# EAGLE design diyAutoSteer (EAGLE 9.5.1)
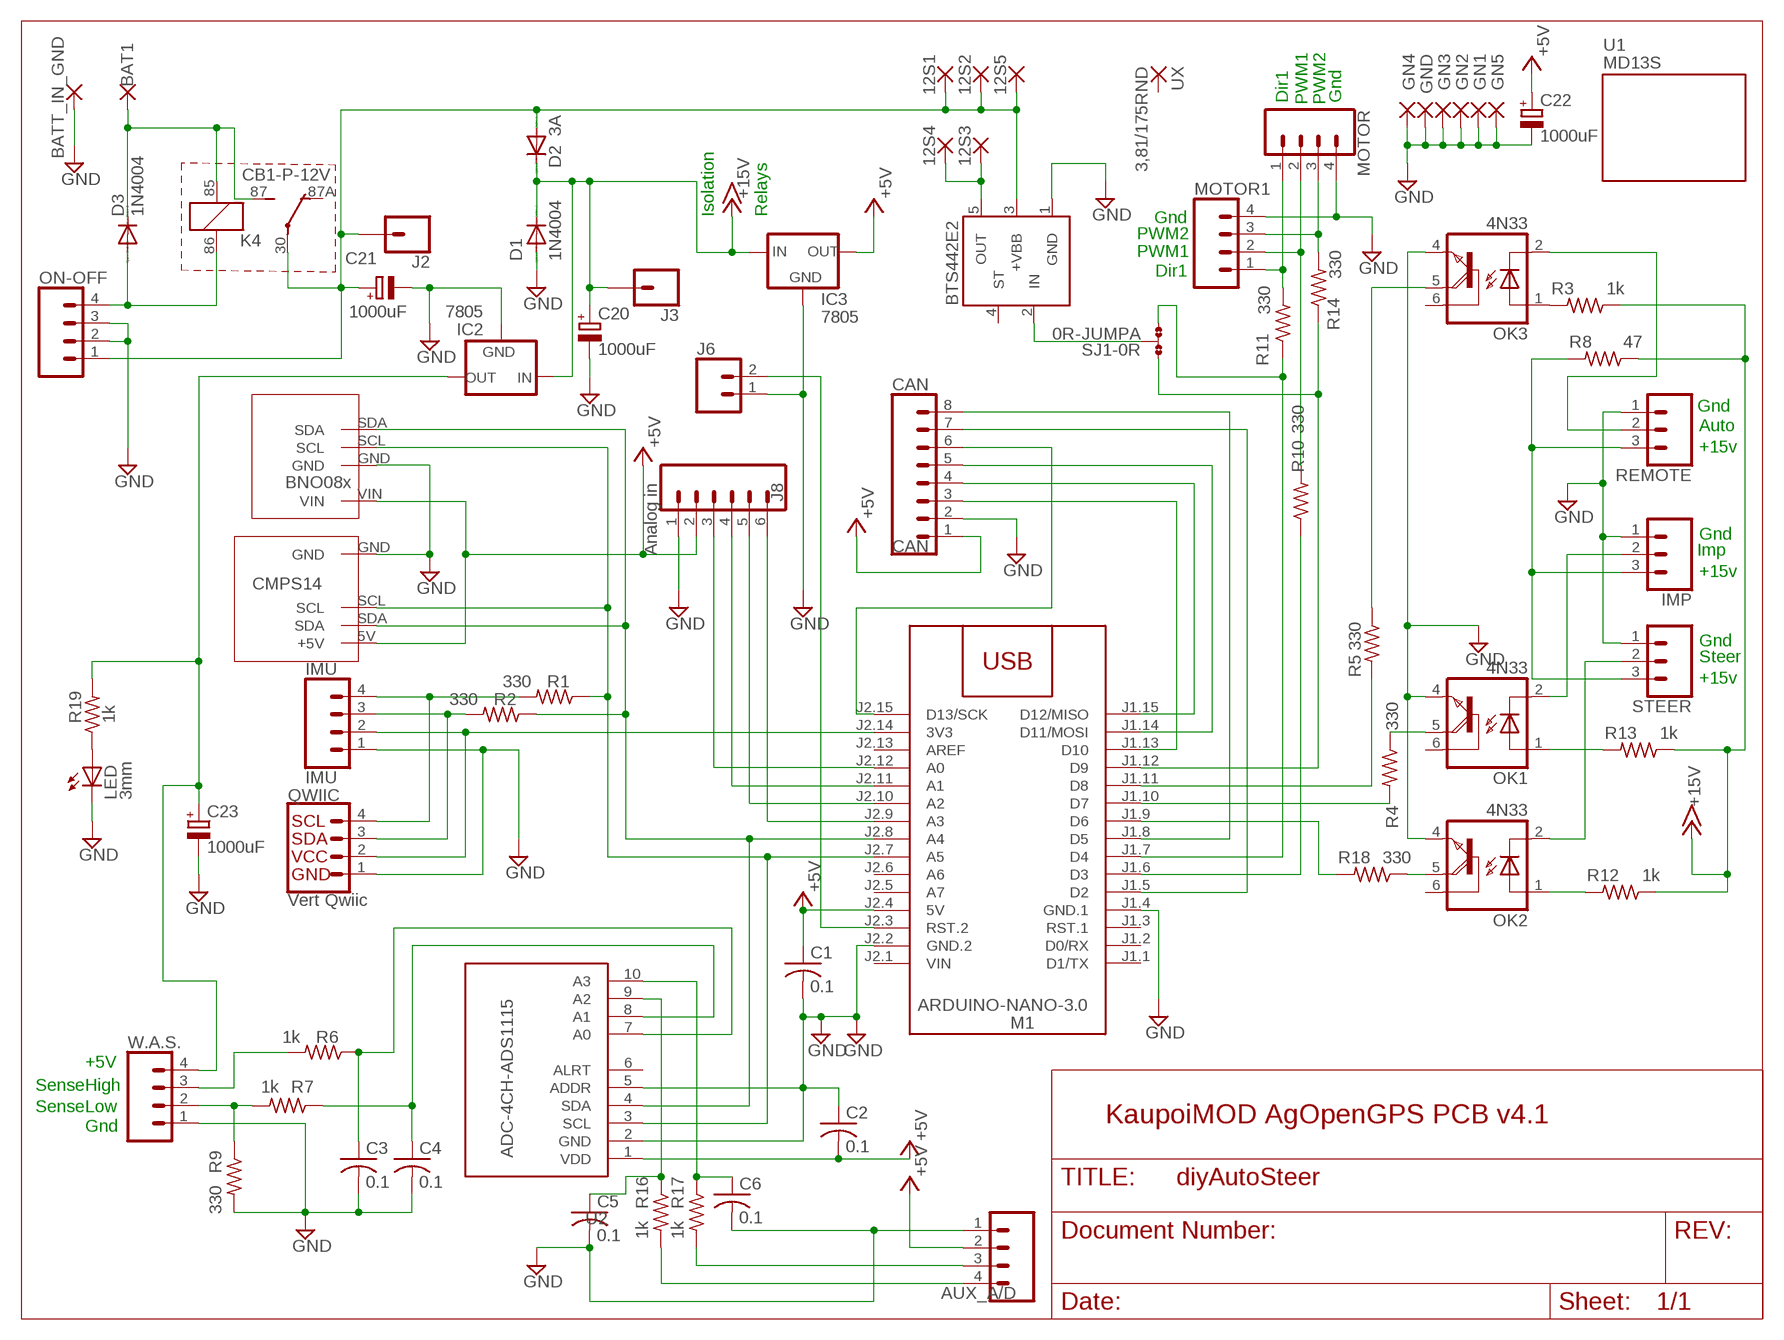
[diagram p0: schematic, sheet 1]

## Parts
12S1  3,81/1,65  [3,81/1,65]
12S2  3,81/1,65  [3,81/1,65]
12S3  3,81/1,65  [3,81/1,65]
12S4  3,81/1,65  [3,81/1,65]
12S5  3,81/1,65  [3,81/1,65]
AUX_A/D  CONN_04LONGPADS  [1X04_LONGPADS]
BAT1  3,81/1,65  [3,81/1,65]
BATT_IN_GND  3,81/1,65  [3,81/1,65]
C1  0.1  C-US025-025X050  [C025-025X050]
C2  0.1  C-US025-025X050  [C025-025X050]
C3  0.1  C-US025-025X050  [C025-025X050]
C4  0.1  C-US025-025X050  [C025-025X050]
C5  0.1  C-US025-025X050  [C025-025X050]
C6  0.1  C-US025-025X050  [C025-025X050]
C20  1000uF  CPOL-EUE5-13  [E5-13]
C21  1000uF  CPOL-EUE5-13  [E5-13]
C22  1000uF  CPOL-EUE5-13  [E5-13]
C23  1000uF  CPOL-EUE5-13  [E5-13]
CAN  CAN  CONN_08NO_SILK_FEMALE_PTH  [1X08_NO_SILK]
D1  1N4004  [DO41-10]
D2  3A  DIODE-DO27-15  [DO27-15]
D3  1N4004  [DO41-10]
GN1  3,81/1,65  [3,81/1,65]
GN2  3,81/1,65  [3,81/1,65]
GN3  3,81/1,65  [3,81/1,65]
GN4  3,81/1,65  [3,81/1,65]
GN5  3,81/1,65  [3,81/1,65]
GND  3,81/1,65  [3,81/1,65]
IC2  7805  78XXS  [78XXS]
IC3  7805  78XXS  [78XXS]
IMP  CONN_03LONGPADS  [1X03_LONGPADS]
IMU  IMU  CONN_04LONGPADS  [1X04_LONGPADS]
J2  CONN_01  [1X01]
J3  CONN_01  [1X01]
J6  CONN_02PTH3  [1X02_LONGPADS]
J8  Analog in  CONN_06NO_SILK_NO_POP  [1X06_NO_SILK]
K4  CB1-P-12V  [CB1]
LED  3mm  LED3MM  [LED3MM]
M1  ARDUINO-NANO-3.0  [ARDUINO-NANO-3.0]
MOTOR  CONN_04LONGPADS  [1X04_LONGPADS]
MOTOR1  CONN_04LONGPADS  [1X04_LONGPADS]
OK1  4N33  [DIL06]
OK2  4N33  [DIL06]
OK3  4N33  [DIL06]
ON-OFF  CONN_04LONGPADS  [1X04_LONGPADS]
QWIIC  Vert Qwiic  QWIIC_CONNECTOR  [JST04_1MM_VERT]
R1  330  R-US_0309/12  [0309/12]
R2  330  R-US_0309/12  [0309/12]
R3  1k  R-US_0309/12  [0309/12]
R4  330  R-US_0309/12  [0309/12]
R5  330  R-US_0309/12  [0309/12]
R6  1k  R-US_0309/12  [0309/12]
R7  1k  R-US_0309/12  [0309/12]
R8  47  R-US_0309/12  [0309/12]
R9  330  R-US_0309/12  [0309/12]
R10  330  R-US_0309/12  [0309/12]
R11  330  R-US_0309/12  [0309/12]
R12  1k  R-US_0309/12  [0309/12]
R13  1k  R-US_0309/12  [0309/12]
R14  330  R-US_0309/12  [0309/12]
R16  1k  R-US_0309/12  [0309/12]
R17  1k  R-US_0309/12  [0309/12]
R18  330  R-US_0309/12  [0309/12]
R19  1k  R-US_0309/12  [0309/12]
REMOTE  CONN_03LONGPADS  [1X03_LONGPADS]
SJ1  0R-JUMPA  [A0R-JMP]
STEER  CONN_03LONGPADS  [1X03_LONGPADS]
U1  MD13S  [MD13S]
U2  ADC-4CH-ADS1115  [ADC-4CH-ADS1115]
U3  BTS442E2  [TO220-5]
U4  CMPS14  [CMPS14]
U5  BNO085  [BNO085]
UX  3,81/175RND  [3,81/1,75RND]
W.A.S.  CONN_04LONGPADS  [1X04_LONGPADS]

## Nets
+5V: AUX_A/D.2 C1.1 C2.2 C22.+ CAN.1 IC3.OUT J8.2 M1.J2.4(5V) U2.1(VDD) U4.5V(+5V) U5.VIN
+15V: C20.+ D1.C D2.C IC2.IN IC3.IN J3.1 R3.1 R8.1 R12.1 R13.1
BATT: BAT1.P$1(P) D3.C K4.85 K4.87(2:S)
DIR: MOTOR1.1 MOTOR.1 R11.2
GND: AUX_A/D.1 BATT_IN_GND.P$1(P) C1.2 C2.1 C3.2 C4.2 C5.2 C6.2 C20.- C21.- C22.- C23.- CAN.2 D1.A GN1.P$1(P) GN2.P$1(P) GN3.P$1(P) GN4.P$1(P) GN5.P$1(P) GND.P$1(P) IC2.GND IC3.GND IMP.1 IMU.1 J6.1 J8.1 LED.K(C) M1.J1.4(GND.1) M1.J2.2(GND.2) MOTOR1.4 MOTOR.4 OK1.4(E) OK2.4(E) OK3.4(E) ON-OFF.2 ON-OFF.3 QWIIC.1 R9.2 REMOTE.1 STEER.1 U2.2(GND) U2.5(ADDR) U3.1(GND) U4.GND U5.GND W.A.S..1
N$1: IMU.2 M1.J2.14(3V3) QWIIC.2
N$2: R7.2 R9.1 W.A.S..2
N$3: IMP.3 R8.2 REMOTE.3 STEER.3
N$4: M1.J1.6(D3) R10.1
N$5: M1.J1.7(D4) R11.1 SJ1.3
N$6: CAN.7 M1.J1.5(D2)
N$7: J6.2 M1.J2.3(RST.2)
N$8: R6.2 W.A.S..3
N$9: CAN.8 M1.J1.8(D5)
N$10: J8.4 M1.J2.11(A1)
N$11: M1.J1.12(D9) R14.1 SJ1.1
N$12: IMU.3 QWIIC.3 R2.2
N$13: IMU.4 QWIIC.4 R1.2
N$14: J8.5 M1.J2.10(A2)
N$15: J8.6 M1.J2.9(A3)
N$16: LED.A R19.1
N$17: CAN.6 M1.J2.15(D13/SCK)
N$18: AUX_A/D.3 R17.2
N$19: OK1.5(COL) R4.1
N$20: C3.1 R6.1 U2.7(A0)
N$21: CAN.5 M1.J1.14(D11/MOSI)
N$22: OK2.2(C) STEER.2
N$23: M1.J1.11(D8) R5.2
N$24: D3.A K4.86 ON-OFF.4
N$25: OK2.1(A) R12.2
N$26: OK3.1(A) R3.2
N$27: M1.J1.10(D7) R4.2
N$28: OK3.2(C) REMOTE.2
N$29: IMP.2 OK1.2(C)
N$30: J8.3 M1.J2.12(A0)
N$31: M1.J1.9(D6) R18.2
N$32: OK1.1(A) R13.2
N$33: CAN.4 M1.J1.15(D12/MISO)
N$34: OK3.5(COL) R5.1
N$35: C6.1 R17.1 U2.10(A3)
N$36: C5.1 R16.1 U2.9(A2)
N$37: CAN.3 M1.J1.13(D10)
N$38: M1.J2.7(A5) R1.1 U2.3(SCL) U4.SCL U5.SCL
N$39: OK2.5(COL) R18.1
N$40: 12S3.P$1(P) 12S4.P$1(P) U3.5(OUT)
N$41: SJ1.2 U3.2(IN)
N$44: C4.1 R7.1 U2.8(A1)
N$47: AUX_A/D.4 R16.2
PWM1: MOTOR1.2 MOTOR.2 R10.2
PWM2: MOTOR1.3 MOTOR.3 R14.2
SDA: M1.J2.8(A4) R2.1 U2.4(SDA) U4.SDA U5.SDA
SW_RAW: 12S1.P$1(P) 12S2.P$1(P) 12S5.P$1(P) C21.+ D2.A J2.1 K4.30(2:P) ON-OFF.1 U3.3(+VBB)
V+WAS: C23.+ IC2.OUT R19.2 W.A.S..4
Unconnected: K4.87A(2:O) M1.J1.1(D1/TX) M1.J1.2(D0/RX) M1.J1.3(RST.1) M1.J2.5(A7) M1.J2.6(A6) M1.J2.13(AREF) OK1.6(B) OK2.6(B) OK3.6(B) U2.6(ALRT) U3.4(ST) UX.P$1(P)

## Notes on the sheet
- Dir1 | PWM1 | PWM2 | Gnd
- Gnd
- Isolation | Relays
- PWM2
- PWM1
- Dir1
- Gnd
- Auto
- +15v
- Gnd
- Imp
- +15v
- Gnd
- Steer
- +15v
- +5V
- Sense | High
- Sense | Low
- KaupoiMOD AgOpenGPS PCB v4.1
- Gnd

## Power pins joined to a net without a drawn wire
VIN: M1.J2.1(VIN)

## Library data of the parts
12S1-12S5 BAT1 BATT_IN_GND GN1-GN5 GND = wirepad:3,81/1,65: 3,81/1,65
AUX_A/D IMU MOTOR MOTOR1 ON-OFF W.A.S. = SparkFun-Connectors:CONN_04: Multi connection point. Often used as Generic Header-pin footprint for 0.1 inch spaced/style header connections On any of the 0.1 inch spaced packages, you can populate with these: Break Away Headers - Straight (PRT-00116) Break Away Male Headers - Right Angle (PRT-00553) Female Headers (PRT-00115)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; PROD_ID: CONN-09696
C1-C6 = rcl:C-US: CAPACITOR, American symbol
C20 = rcl:CPOL-EU: POLARIZED CAPACITOR, European symbol; SPICEPREFIX: C
C21-C23 = rcl:CPOL-EU: POLARIZED CAPACITOR, European symbol
CAN = SparkFun-Connectors:CONN_08: Multi connection point. Often used as Generic Header-pin footprint for 0.1 inch spaced/style header connections On any of the 0.1 inch spaced packages, you can populate with these: Break Away Headers - Straight (PRT-00116) Break Away Male Headers - Right Angle (PRT-00553) Female Headers (PRT-00115)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; PROD_ID: CONN-08438
D1 D3 = diode:1N4004: DIODE
D2 = diode:DIODE-: DIODE
IC2 IC3 = v-reg:78XXS: VOLTAGE REGULATOR
IMP REMOTE STEER = SparkFun-Connectors:CONN_03: Multi connection point. Often used as Generic Header-pin footprint for 0.1 inch spaced/style header connections On any of the 0.1 inch spaced packages, you can populate with these: Break Away Headers - Straight (PRT-00116) Break Away Male Headers - Right Angle (PRT-00553) Female Headers (PRT-00115)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
J2 J3 = SparkFun-Connectors:CONN_01: Single connection point. Often used as Generic Header-pin footprint for 0.1 inch spaced/style header connections
J6 = SparkFun-Connectors:CONN_02: Multi connection point. Often used as Generic Header-pin footprint for 0.1 inch spaced/style header connections
J8 = SparkFun-Connectors:CONN_06: Multi connection point. Often used as Generic Header-pin footprint for 0.1 inch spaced/style header connections On any of the 0.1 inch spaced packages, you can populate with these: Break Away Headers - Straight (PRT-00116) Break Away Male Headers - Right Angle (PRT-00553) Female Headers (PRT-00115)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
K4 = relay:CB1*: HIGH POWER AUTOMOTIVE RELAY Form C NAiS Source: http://www.mew-europe.com/.. en_ds_61202_0000.pdf; MF: AROMAT/ MATSUSHITA; MPN: CB1-P-12V; OC_FARNELL: unknown; OC_NEWARK: 52F9201
LED = led:LED: LED
M1 = diy-modules:ARDUINO-NANO-3.0: Arduino Nano 3.0 and compatible devices More details available here: https://www.arduino.cc/en/Main/ArduinoBoardNano Click here to find device on ebay.com
OK1-OK3 = optocoupler:4N33: MOTOROLA OPTO COUPLER; MF: VISHAY/TELEFUNKEN; MPN: 4N33; OC_FARNELL: 1469601; OC_NEWARK: 88K1390
QWIIC = SparkFun-Connectors:QWIIC_CONNECTOR: SparkFun I2C Standard Qwiic Connector An SMD 1mm pitch JST connector makes it easy and quick (get it? Qwiic?) to connect I2C devices to each other. The Qwiic system enables fast and solderless connection between popular platforms and various sensors and actuators. We carry 200mm, 100mm, 50mm, and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; PROD_ID: CONN-14483; VALUE: Vertical Qwiic Connector
R1-R14 R16-R19 = rcl:R-US_: RESISTOR, American symbol
SJ1 = jump-0r-smd:0R-JUMP: SMD 0R 0805 Jumper
U1 = cytronMD13Sholes:MD13S: 13Amp DC Motor Driver (MD13S); CYTRON-PC: MD13S; DESC: 13Amp DC Motor Driver - GROVE Compatible; MF: Cytron; MPN: MD13S
U2 = diy-modules:ADC-4CH-ADS1115: 4 Channel 16-Bit Analog-to-Digital Converter based on ADS1115 chip Arduino ADS1115 Getting Started Tutorial is available here: http://henrysbench.capnfatz.com/henrys-bench/arduino-voltage-measurements/arduino-ads1115-module-getting-started-tutorial/ ADS1115 datasheet is available here: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
U3 = v-reg-3:BTS442E2
U4 = IMU:CMPS14: CMPS14
U5 = IMU:BNO085
UX = wirepad:3,81/175RND

## Module MOTOR_CONTROLLER
Ports: 

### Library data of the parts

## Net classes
0 default: clearance 0.205 mm

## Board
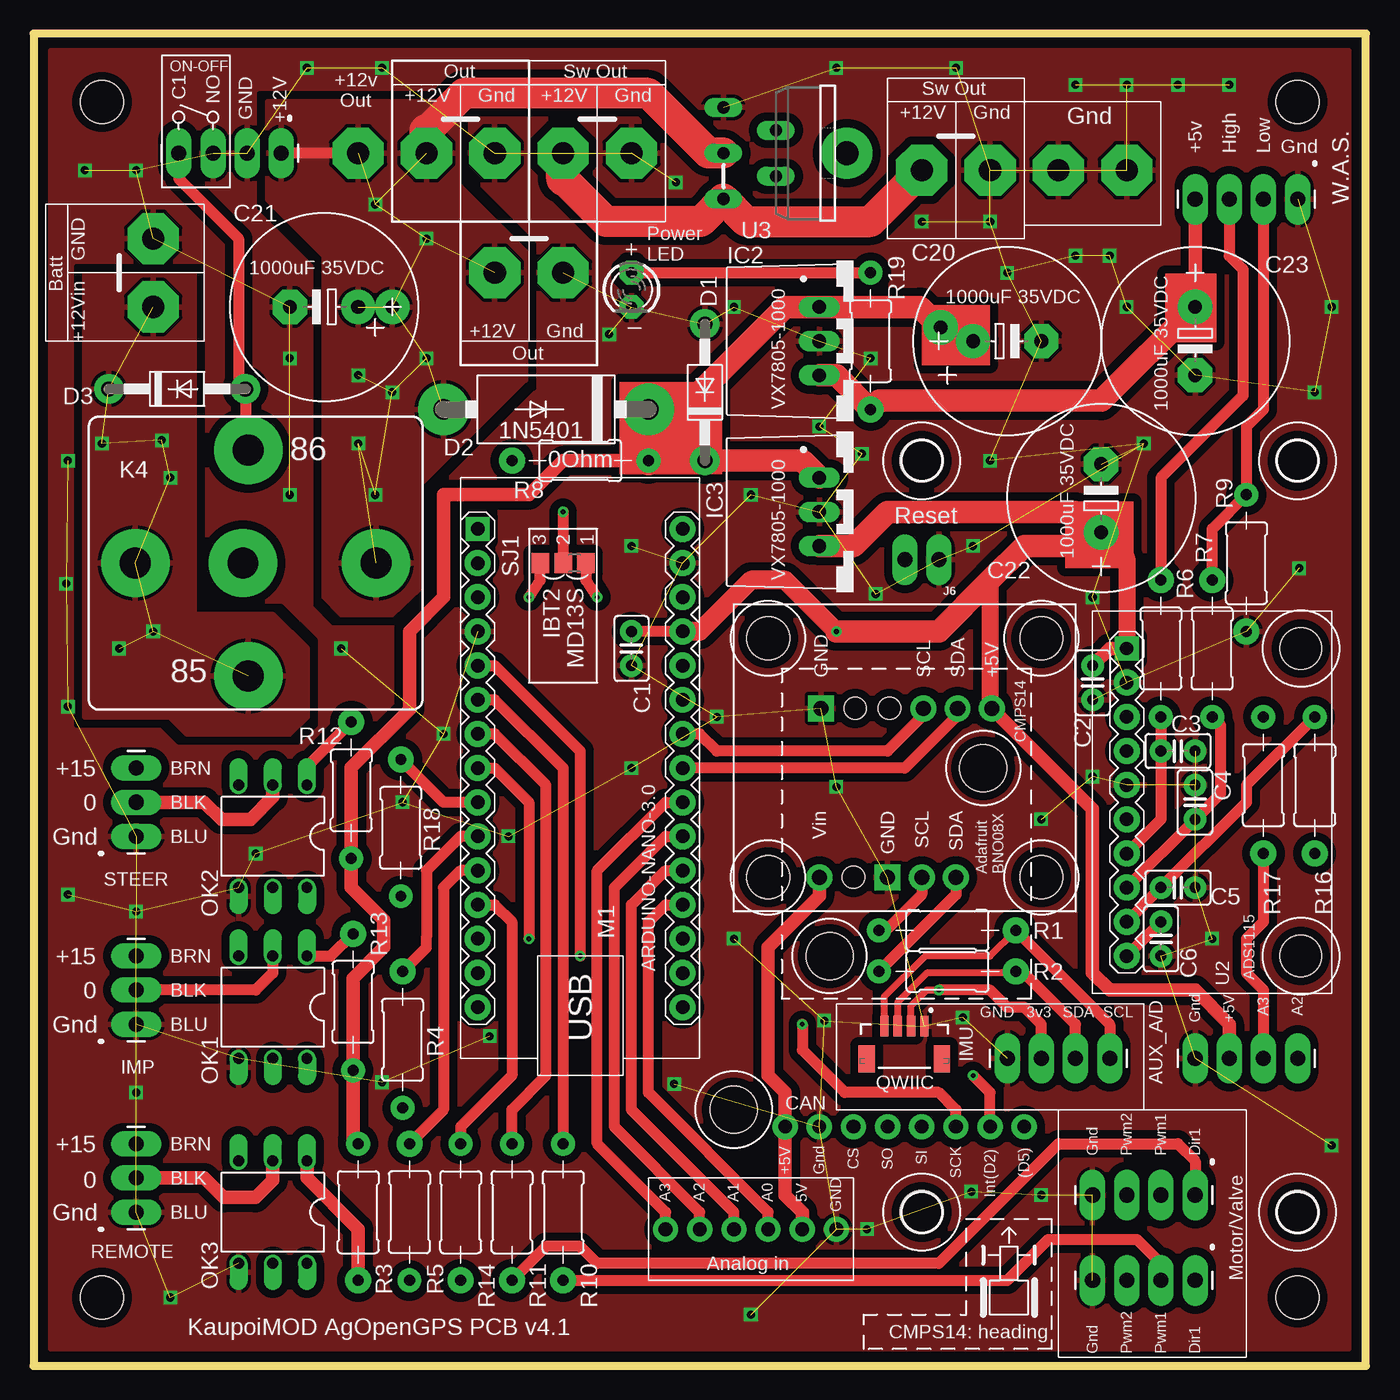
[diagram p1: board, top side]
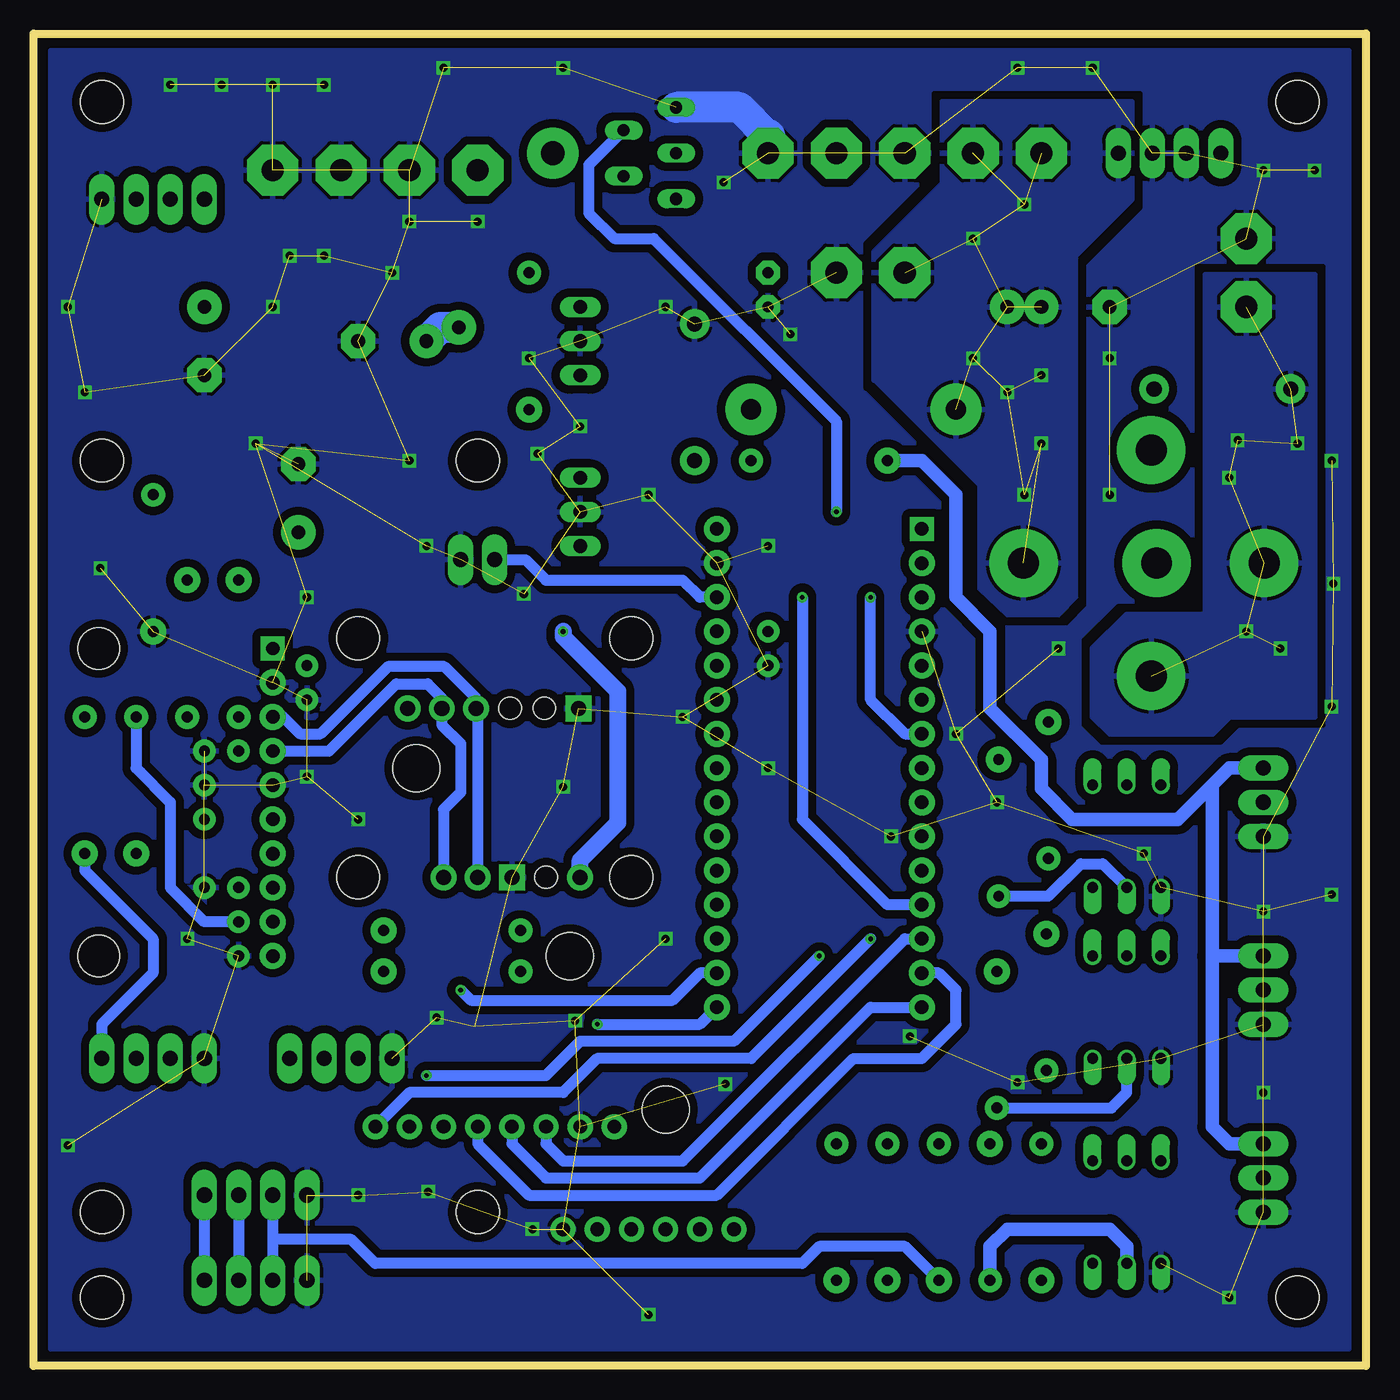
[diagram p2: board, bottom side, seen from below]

Size 99.06 x 99.06 mm. Coordinates in mm from the lower left corner, seen from the top.
Outline: 0,0 99.06,0 99.06,99.06 0,99.06 0,0
Copper layers (1*16): Top 0.035mm / dielectric 1.5mm / Bottom 0.035mm
Design rules "default *": minimum track width 16mil, minimum drill 0.35mm, track to track 6mil, track to pad 6mil, pad to pad 6mil, via to via 6mil, smd to smd 6mil, copper to edge 8mil, drill to drill 6mil, minimum pad ring 10mil, minimum via ring 8mil, stop-mask expansion 4mil, vias tented up to drill 0mil, thermal gap 10mil
Holes 3.2 mm at 5.08,5.08 93.98,5.08 5.08,93.98 93.98,93.98
Holes 3.5 mm at 52.07,19.05

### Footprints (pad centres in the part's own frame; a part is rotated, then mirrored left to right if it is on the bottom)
3,81/1,65 = drill 1.651 pad 3.81 octagon: P$1 0,0
1X04_LONGPADS = drill 1.118 pad 1.88 long: 1 0,0; 2 2.54,0; 3 5.08,0; 4 7.62,0
C025-025X050 = drill 0.813 pad 1.676: 1 -1.27,0; 2 1.27,0
E5-13 = drill 1.016 pad 2.54: + -2.54,0 | drill 1.016 pad 2.54 octagon: - 2.54,0
1X08_NO_SILK = drill 1.016 pad 1.88: 1 0,0; 2 2.54,0; 3 5.08,0; 4 7.62,0; 5 10.16,0; 6 12.7,0; 7 15.24,0; 8 17.78,0
DO41-10 = drill 1.118 pad 2.184: A 5.08,0; C -5.08,0
DO27-15 = drill 1.499 pad 3.81: A 7.62,0; C -7.62,0
78XXS = drill 1.016 long: GND 0,-2.54; IN -2.54,-2.54; OUT 2.54,-2.54
1X03_LONGPADS = drill 1.118 pad 1.88 long: 1 0,0; 2 2.54,0; 3 5.08,0
1X01 = drill 1.016 pad 2.54: 1 0,0
1X02_LONGPADS = drill 1.118 pad 1.88 long: 1 0,0; 2 2.54,0
1X06_NO_SILK = drill 1.016 pad 1.88: 1 0,0; 2 2.54,0; 3 5.08,0; 4 7.62,0; 5 10.16,0; 6 12.7,0
CB1 = drill 2.3 pad 5.08: 30 8.95,0; 85 -0.55,-8.4; 86 -0.55,8.4; 87 -8.95,0; 87A -0.95,0
LED3MM = drill 0.813 pad 1.778 octagon: A -1.27,0; K 1.27,0
ARDUINO-NANO-3.0 = drill 1 pad 1.778 square: J1.1 17.78,7.62 | drill 1 pad 1.93: J1.2 15.24,7.62; J1.3 12.7,7.62; J1.4 10.16,7.62; J1.5 7.62,7.62; J1.6 5.08,7.62; J1.7 2.54,7.62; J1.8 0,7.62; J1.9 -2.54,7.62; J1.10 -5.08,7.62; J1.11 -7.62,7.62; J1.12 -10.16,7.62; J1.13 -12.7,7.62; J1.14 -15.24,7.62; J1.15 -17.78,7.62; J2.1 17.78,-7.62; J2.2 15.24,-7.62; J2.3 12.7,-7.62; J2.4 10.16,-7.62; J2.5 7.62,-7.62; J2.6 5.08,-7.62; J2.7 2.54,-7.62; J2.8 0,-7.62; J2.9 -2.54,-7.62; J2.10 -5.08,-7.62; J2.11 -7.62,-7.62; J2.12 -10.16,-7.62; J2.13 -12.7,-7.62; J2.14 -15.24,-7.62; J2.15 -17.78,-7.62
DIL06 = drill 0.813 offset: 1 -2.54,-3.81; 2 0,-3.81; 3 2.54,-3.81; 4 2.54,3.81; 5 0,3.81; 6 -2.54,3.81
JST04_1MM_VERT = smd 0.6 x 1.55: 1 -1.478,0.775; 2 -0.478,0.775; 3 0.522,0.775; 4 1.522,0.775 | smd 1.2 x 2: NC1 -2.778,3.2; NC2 2.822,3.2
0309/12 = drill 0.813 pad 1.778: 1 -5.08,0 | drill 0.813 pad 1.93: 2 5.08,0
A0R-JMP = smd 1.5 x 1.3: 1 0,1.7; 2 0,0; 3 0,-1.7
MD13S = hole 3.2: 2.54,30.48; 2.54,2.54; 58.42,2.54; 58.42,30.48
ADC-4CH-ADS1115 = drill 1 pad 1.778 square: 1 -6.35,11.43 | drill 1 pad 1.93: 2 -6.35,8.89; 3 -6.35,6.35; 4 -6.35,3.81; 5 -6.35,1.27; 6 -6.35,-1.27; 7 -6.35,-3.81; 8 -6.35,-6.35; 9 -6.35,-8.89; 10 -6.35,-11.43 | hole 3.1: 6.604,11.43; 6.604,-11.43
TO220-5 = drill 0.9 long: 1 -3.4,-8.4; 2 -1.7,-4.5; 3 0,-8.4; 4 1.7,-4.5; 5 3.4,-8.4
CMPS14 = drill 1.118 pad 1.93: 5V 10.16,-6.35; SCL 10.16,-1.27; SDA 10.16,-3.81 | drill 1.118 pad 1.93 square: GND 10.16,6.35 | hole 3.5: 5.715,-5.715; -8.255,5.715 | hole 1.676: 10.16,1.27; 10.16,3.81
BNO085 = drill 1.118 pad 1.93 square: GND 8.89,-1.27 | drill 1.118 pad 1.93: SCL 8.89,1.27; SDA 8.89,3.81; VIN 8.89,-6.35 | hole 3.2: 8.89,10.16; 8.89,-10.16; -8.89,-10.16; -8.89,10.16 | hole 1.651: 8.89,-3.81
3,81/1,75RND = drill 1.75 pad 3.81: P$1 0,0

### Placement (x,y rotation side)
12S1  29.21,90.17 0 top
12S2  24.13,90.17 0 top
12S3  39.37,90.17 0 top
12S4  66.04,88.9 0 top
12S5  34.29,81.28 0 top
AUX_A/D  86.36,22.86 0 top
BAT1  8.89,78.74 0 top
BATT_IN_GND  8.89,83.82 0 top
C1  44.45,53.34 270 top
C2  78.74,50.8 90 top
C3  85.09,45.72 0 top
C4  86.36,41.91 90 top
C5  85.09,35.56 0 top
C6  83.82,31.75 270 top
C20  72.39,76.2 0 top
C21  21.59,78.74 180 top
C22  79.38,64.52 90 top
C23  86.36,76.2 270 top
CAN  55.88,17.78 0 top
D1  49.91,72.39 90 top
D2  38.1,71.12 180 top
D3  10.67,72.64 0 top
GN1  34.29,90.17 0 top
GN2  71.12,88.9 0 top
GN3  81.28,88.9 0 top
GN4  44.45,90.17 0 top
GN5  39.37,81.28 0 top
GND  76.2,88.9 0 top
IC2  60.96,76.2 270 top
IC3  60.96,63.5 270 top
IMP  7.62,25.4 90 top
IMU  72.39,22.86 0 top
J2  26.67,78.74 0 top
J3  67.44,77.22 0 top
J6  67.31,59.94 180 top
J8  59.69,10.16 180 top
K4  16.51,59.69 0 top
LED  44.45,80.01 270 top
M1  40.64,44.45 90 top
MOTOR  86.36,6.35 180 top
MOTOR1  86.36,12.7 180 top
OK1  17.78,26.67 180 top
OK2  17.78,39.37 180 top
OK3  17.78,11.43 180 top
ON-OFF  18.41,90.17 180 top
QWIIC  64.77,26.04 180 top
R1  67.95,32.38 0 top
R2  67.95,29.34 0 top
R3  24.13,11.43 270 top
R4  27.43,24.26 90 top
R5  27.94,11.43 90 top
R6  83.82,53.34 90 top
R7  87.63,53.34 90 top
R8  40.64,67.31 180 top
R9  90.17,59.69 270 top
R10  39.37,11.43 270 top
R11  35.56,11.43 270 top
R12  23.62,42.8 90 top
R13  23.75,27.05 90 top
R14  31.75,11.43 270 top
R16  95.25,43.18 270 top
R17  91.44,43.18 270 top
R18  27.3,40.01 90 top
R19  62.23,76.2 270 top
REMOTE  7.62,11.43 90 top
SJ1  39.37,59.69 270 top
STEER  7.62,39.37 90 top
U1  96.52,8.89 90 top
U2  87.63,41.91 0 top
U3  59.69,90.17 270 top
U4  64.9,38.73 90 top
U5  64.77,45.21 270 top
UX  60.45,90.17 0 top
W.A.S.  93.98,86.74 180 top

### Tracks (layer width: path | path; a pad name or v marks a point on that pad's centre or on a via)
+5V  (via drill 0.35)
  Top 0.813: M1.J2.4 C1.1
  Top 1.016: U2.1 80.01,53.34 C2.2 | U4.5V 78.74,41.4 78.74,29.21 80.01,27.94 86.36,27.94 88.9,25.4 AUX_A/D.2 | U5.VIN 58.42,34.92 54.61,31.11 54.61,21.59 55.88,20.32 CAN.1 55.88,12.7 57.15,11.43 J8.2
  Top 1.27: C22.+ 81.28,60.07 U2.1 | 71.12,58.42 71.12,49.02 U4.5V
  Top 1.422: v59.69,54.61 55.88,58.42 53.34,58.42 49.53,54.61 M1.J2.4
  Top 1.676: v59.69,54.61 67.31,54.61 71.12,58.42 73.66,60.96 78.36,60.96 C22.+ 78.99,61.98 77.47,63.5 63.5,63.5 60.96,60.96 IC3.OUT
  Bottom 1.27: v59.69,54.61 59.69,54.23 55.63,50.16 55.63,40.39 58.42,37.59 U5.VIN
+15V
  Top 1.016: R3.1 23.75,16.89 R13.1 23.75,28.83 26.04,31.11 26.04,33.15 23.62,35.56 R12.1 23.62,44.49 27.94,48.81 27.94,54.61 30.48,57.15 30.48,64.77 30.49,64.78 36.84,64.78 39.37,67.31 R8.1 49.53,66.93 D1.C
  Top 1.676: D2.C 45.8,71.2 48.34,71.2 55.88,78.74 IC2.IN 65.91,78.74 J3.1 | R8.1 57.15,67.31 IC3.IN
  Top 2.184: R8.1 D2.C
  Bottom 2.286: J3.1 68.83,77.22 C20.+
BATT  (via drill 0.6)  (8 unrouted)
  other vias: 9.53,68.83 5.08,68.58 8.89,54.61 10.16,66.04 6.35,53.34
  pour Bottom (isolate 0.406): 19.05,46.99 20.32,48.26 20.32,53.34 17.78,55.88 11.94,55.88 11.94,81.15 3.81,81.15 3.81,48.26 10.16,48.26 11.43,46.99
  pour Top (isolate 0.406): 3.81,81.15 3.81,48.26 10.16,48.26 11.43,46.99 19.05,46.99 20.32,48.26 20.32,53.34 17.78,55.88 11.94,55.88 11.94,81.15
DIR
  Top 0.813: R11.2 38.1,8.89 40.64,8.89 41.91,7.62 67.31,7.62 76.2,16.51 85.09,16.51 86.36,15.24 MOTOR1.1
  Bottom 0.813: MOTOR1.1 MOTOR.1
GND  (via drill 0.6)  (107 unrouted)
  Bottom 2.286: 44.45,91.44 46.58,93.57 U3.1
  Bottom 2.54: GN4.P$1 44.45,91.44
  other vias: 20.32,96.52 7.62,88.9 42.8,76.71 59.69,96.52 96.52,78.74 47.75,88.01 88.9,95.25 33.91,24.51 81.28,78.74 95.25,72.39 62.23,74.93 61.59,67.82 58.42,69.85 53.34,64.77 27.43,41.91 30.48,46.99 52.07,78.74 66.04,85.09 72.39,81.28 71.12,85.09 77.47,82.55 2.54,67.31 2.54,49.02 7.62,20.32 94.11,59.31 53.34,3.81 47.62,20.95 78.74,57.15 69.09,25.91 3.81,88.9 25.91,96.52 19.05,74.93 19.05,64.77 22.86,53.34 2.41,58.17 7.62,33.78 16.51,38.1 69.85,60.96 81.28,95.25 44.45,44.45 44.45,60.96 85.09,95.25 80.01,82.55 62.61,57.4 71.12,67.31 96.52,16.38 69.72,12.95 78.74,43.81 10.16,5.08 52.07,31.75 82.55,68.58 59.69,43.05 50.8,48.26 87.63,31.75 61.98,10.16 2.54,35.05 77.47,95.25 74.93,12.7 25.91,21.08 58.8,25.65 74.93,40.64 68.58,96.52 35.31,39.37
  pour Bottom (isolate 0.61, rank 2): 1.27,97.79 1.27,1.27 97.79,1.27 97.79,97.79
  pour Top (isolate 0.61, rank 2): 1.27,97.79 1.27,1.27 97.79,1.27 97.79,97.79
N$1  (via drill 0.35)
  Top 0.508: QWIIC.2 65.25,26.77 66.42,27.94 v67.31,27.94
  Top 0.813: IMU.2 74.93,25.4 73.66,26.67 72.39,26.67 71.12,27.94 v67.31,27.94
  Bottom 0.813: M1.J2.14 49.53,29.21 51.56,27.18 66.55,27.18 v67.31,27.94
N$2
  Top 0.813: R7.2 87.63,62.23 R9.1 90.17,69.85 91.44,71.12 W.A.S..2
N$3
  Bottom 1.016: 11.43,43.18 10.16,44.45 STEER.3 | 11.43,43.18 11.43,30.48 | IMP.3 11.43,30.48 | 11.43,30.48 11.43,17.78 10.16,16.51 REMOTE.3 | 11.43,43.18 13.97,40.64 21.84,40.64 24.13,42.93 24.13,45.09 27.94,48.9 27.94,54.61 30.48,57.15 30.48,64.77 33.02,67.31 R8.2
N$4
  Top 0.813: R10.1 39.37,44.45 34.29,49.53 M1.J1.6
N$5  (via drill 0.35)
  Top 0.813: R11.1 35.56,19.05 38.1,21.59 38.1,43.18 34.29,46.99 M1.J1.7 | SJ1.3 37.67,58.42 v36.83,57.15
  Bottom 0.813: M1.J1.7 34.29,46.99 36.83,49.53 v36.83,57.15
N$6  (via drill 0.35)
  Top 0.813: M1.J1.5 34.29,52.07 40.64,45.72 v40.64,30.48 | CAN.7 71.12,20.32 v69.85,21.59
  Bottom 0.813: v40.64,30.48 46.99,24.13 58.42,24.13 60.96,21.59 v69.85,21.59
N$7
  Bottom 0.813: J6.2 62.48,59.94 60.96,58.42 50.8,58.42 49.53,57.15 M1.J2.3
N$8
  Top 0.813: R6.2 83.82,66.04 89.92,72.14 89.92,81.53 88.9,82.55 W.A.S..3
N$9  (via drill 0.35)
  Top 0.813: M1.J1.8 34.29,44.45 36.83,41.91 v36.83,31.75
  Bottom 0.813: v36.83,31.75 45.72,22.86 57.15,22.86 59.69,20.32 71.12,20.32 CAN.8
N$10
  Top 0.813: J8.4 52.07,11.43 44.45,19.05 44.45,34.29 46.99,36.83 M1.J2.11
N$11  (via drill 0.35)
  Top 0.813: M1.J1.12 34.29,34.29 35.56,33.02 35.56,21.59 31.75,17.78 R14.1 | SJ1.1 41.07,58.42 v41.91,57.15
  Bottom 0.813: v41.91,57.15 41.91,40.64 35.56,34.29 M1.J1.12
N$12
  Top 0.508: R2.2 72.9,29.21 66.42,29.21 64.23,27.02 64.23,25.27 QWIIC.3
  Top 0.813: IMU.3 77.47,25.4 73.53,29.34 R2.2
N$13
  Top 0.508: QWIIC.4 63.23,25.27 63.23,27.42 66.29,30.48 71.12,30.48 R1.2
  Top 0.813: R1.2 80.01,25.4 80,22.87 IMU.4
N$14
  Top 0.813: J8.5 49.53,11.43 43.18,17.78 43.18,35.56 46.99,39.37 M1.J2.10
N$15
  Top 0.813: J8.6 46.99,11.43 41.91,16.51 41.91,36.83 46.99,41.91 M1.J2.9
N$16
  Top 0.813: LED.A R19.1
N$17  (via drill 0.35)
  Top 0.813: CAN.6 68.58,19.05 67.31,20.32 60.32,20.32 57.15,23.5 v57.15,25.4
  Bottom 0.813: M1.J2.15 49.53,25.4 v57.15,25.4
N$18
  Top 0.813: R17.2 91.44,33.02 90.17,31.75 90.17,29.21 91.44,27.94 AUX_A/D.3
N$19
  Bottom 0.813: R4.1 18.92,19.18 17.78,20.32 OK1.5
N$20
  Top 0.813: U2.7 83.82,40.64 C3.1 R6.1
N$21
  Bottom 0.813: CAN.5 66.04,16.51 62.23,12.7 48.26,12.7 38.1,22.86 33.02,22.86 30.48,25.4 30.48,27.94 31.75,29.21 M1.J1.14
N$22
  Top 1.016: OK2.2 17.78,42.29 16.13,40.64 13.97,40.64 12.7,41.91 STEER.2
N$23
  Top 0.813: M1.J1.11 31.75,36.83 30.48,35.56 30.48,19.05 R5.2
N$24
  Top 0.813: K4.86 15.75,68.3 D3.A 15.24,73.15 15.24,83.82 10.79,88.27 ON-OFF.4
N$25
  Top 0.813: R12.2 20.32,44.58 OK2.1
N$26
  Top 1.016: OK3.1 20.32,13.97 24.13,10.16 R3.2
N$27
  Top 0.813: M1.J1.10 31.75,39.37 29.21,36.83 29.21,31.88 29.21,31.11 R4.2
N$28
  Top 1.016: OK3.2 17.78,13.79 16.5,12.52 14.14,12.53 12.7,13.97 REMOTE.2
N$29
  Top 0.813: OK1.2 17.78,29.21 16.51,27.94 IMP.2
N$30
  Top 0.813: J8.3 54.61,11.43 45.72,20.32 45.72,33.02 46.99,34.29 M1.J2.12
N$31
  Top 0.813: M1.J1.9 30.48,41.91 R18.2
N$32
  Top 0.813: OK1.1 22.1,30.48 R13.2
N$33
  Bottom 0.813: CAN.4 63.5,16.51 60.96,13.97 49.53,13.97 36.83,26.67 M1.J1.15
N$34
  Bottom 1.016: R5.1 27.94,8.89 26.67,10.16 19.05,10.16 17.78,8.89 OK3.5
N$35
  Top 0.813: C6.1 U2.10
  Bottom 0.813: R17.1 91.44,44.45 88.9,41.91 88.9,35.56 86.36,33.02 C6.1
N$36
  Top 0.813: U2.9 C5.1 90.17,41.91 90.17,43.18 R16.1
N$37
  Bottom 0.813: M1.J1.13 34.29,31.75 50.8,15.24 59.69,15.24 60.96,16.51 CAN.3
N$38
  Top 0.813: U4.SCL 66.17,48.39 63.5,45.72 50.8,45.72 49.53,46.99 M1.J2.7 | U5.SCL 66.04,35.05 63.37,32.38 R1.1
  Bottom 0.813: U2.3 80.52,48.26 79.25,46.99 77.72,46.99 72.72,52 68.51,52 66.17,49.66 U4.SCL 66.04,48.77 U5.SCL
N$39
  Bottom 0.813: OK2.5 19.56,37.34 21.21,37.34 23.62,34.92 R18.1
N$40
  Top 2.286: 39.37,88.27 42.54,85.09 49.61,85.09 U3.5 52.97,85.09 62.23,85.09 12S4.P$1
  Top 2.54: 39.37,88.27 12S3.P$1
N$41  (via drill 0.35)
  Top 0.813: v39.37,63.5 SJ1.2
  Bottom 0.813: U3.2 57.78,89.28 57.78,85.72 55.88,83.82 52.96,83.82 39.37,70.23 v39.37,63.5
N$44
  Top 0.813: U2.8 C4.1 88.27,42.55 88.27,47.62 R7.1
N$47
  Bottom 0.813: R16.2 95.25,36.83 90.17,31.75 90.17,29.21 93.98,25.4 AUX_A/D.4
PWM1
  Top 0.813: R10.2 72.39,6.35 75.44,9.4 82.04,9.4 83.82,7.62 MOTOR.2
  Bottom 0.813: MOTOR1.2 MOTOR.2
PWM2
  Bottom 0.813: MOTOR1.3 MOTOR.3 81.28,9.4 75.44,9.4 73.66,7.62 41.91,7.62 40.64,8.89 34.29,8.89 R14.2
SDA
  Top 0.813: U4.SDA 68.71,48.39 64.77,44.45 M1.J2.8 | U5.SDA 68.58,35.05 R2.1
  Bottom 0.813: U2.4 77.09,45.72 72.09,50.72 69.77,50.72 68.71,49.66 U4.SDA 68.71,47.66 67.31,46.26 67.31,42.64 68.58,41.37 U5.SDA
SW_RAW  (via drill 0.6)  (13 unrouted)
  Top 0.813: 12S2.P$1 ON-OFF.1
  Top 2.286: U3.3 50.16,90.17 45.72,94.61 32,94.61 29.21,91.82
  Top 2.54: 12S1.P$1 29.21,91.82
  other vias: 25.4,86.36 29.21,83.82 26.67,72.39 29.21,74.93 25.4,64.77 24.13,73.66 24.13,68.58
  pour Bottom (isolate 0.406): 17.4,93.98 17.4,86.74 21.59,82.55 21.59,57.15 22.86,55.88 26.67,55.88 28.7,57.78 28.7,65.53 36.45,73.28 36.58,73.28 36.58,82.8 31.5,87.88 31.5,93.98
  pour Top (isolate 0.406): 17.4,93.98 17.4,86.74 21.59,82.55 21.59,57.15 22.86,55.88 26.67,55.88 28.7,57.78 28.7,65.53 36.45,73.28 36.58,73.28 36.58,82.8 31.5,87.88 31.5,93.98
V+WAS
  Top 1.016: W.A.S..4 C23.+
  Top 1.676: IC2.OUT 59.69,73.66 R19.2 62.87,71.75 79.38,71.75 C23.+
(copper drawn outside any net)
  shapes: Top area x4

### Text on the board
tPlace: C1 | NO | GND | +12V | Out | Sw Out | +12v / Out | +12V | Gnd | +12V | Gnd | Sw Out | +12V | Gnd | Gnd | +5v | High | Low | Gnd | C21 | + | _ | +12Vin | +12V | Gnd | Out | Reset | 3 | 2 | 1 | IBT2 ( | MD13S ( | +15 | BRN | BLK | 0 | Gnd | BLU | +15 | BRN | BLK | 0 | GND | 3v3 | SDA | SCL | Gnd | +5V | A3 | A2 | Gnd | BLU | BRN | +15 | Int(D2) | Gnd | Pwm2 | Pwm1 | Dir1 | CS | SO | SI | BLK | +5V | Gnd | SCK | (D5) | 0 | A3 | A2 | A1 | A0 | 5V | Gnd | BLU | GND | Analog in | Motor/Valve | KaupoiMOD AgOpenGPS PCB v4.1 | Gnd | Pwm2 | Pwm1 | Dir1
tNames: GND | 1000uF 35VDC | Power / LED | Batt | 1000uF 35VDC | VX7805-1000 | 1000uF 35VDC | 1000uF 35VDC | 1N5401 | 86 | 0Ohm | VX7805-1000 | 85 | ARDUINO-NANO-3.0 | ADS1115 | IMU | R5 | CMPS14: heading

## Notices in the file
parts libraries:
SparkFun-Connectors: Licensing: Creative Commons ShareAlike 4.0 International - https://creativecommons.org/licenses/by-sa/4.0
diy-modules: Released under the Creative Commons Attribution 4.0 International License: http://creativecommons.org/licenses/by/4.0
